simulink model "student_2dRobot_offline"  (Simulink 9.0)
settings: Solver=ode1  StartTime=0.0  StopTime=10  FixedStep=0.002  RelTol=1e-3  AbsTol=1e-6  EnableMultiTasking=on
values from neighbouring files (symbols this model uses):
  K = Am / Beq_v    [d_model_param.m]
  K_AMP = 1    [setup_2d_robot.m]
  K_ENC = 0    [config_srv02.m]
  ki = 0    [setup_2d_robot.m]
  kp = wn^2/K*tau    [d_pv_design.m]    (also in setup_2d_robot.m = 0)
  kv = (-1+2*zeta*wn*tau)/K    [d_pv_design.m]    (also in setup_2d_robot.m = 0)
  Lb_in = 5    [config_2d_robot.m]
  q0 = [0; 0; pi/2; 0]    [setup_2d_robot.m]
  tau = Jeq / Beq_v    [d_model_param.m]
  VMAX_AMP = 0    [config_srv02.m]
  VMAX_DAC = 10    [setup_2d_robot.m]
  wcf = 2 * pi * 50.0    (= 314.159265359)    [setup_2d_robot.m]
  zetaf = 0.9    [setup_2d_robot.m]
undefined symbols (not defined in the file or in its folder): axis_limits, HIL, number_of_trajectories, qc_get_step_size
libraries: quarc_library x4, simulink x2, simulink_extras x2

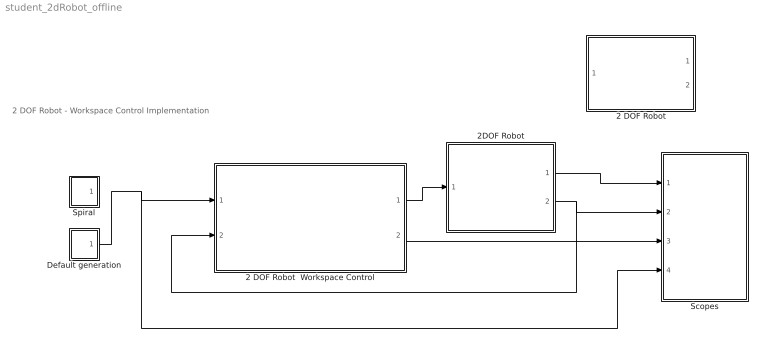
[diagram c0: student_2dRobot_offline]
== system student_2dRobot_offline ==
  note: 2 DOF Robot - Workspace Control Implementation
  2 DOF Robot : Subsystem  Commented=on
  2 DOF Robot  Workspace Control : Subsystem
  2DOF Robot : Subsystem
  Default generation : Subsystem
  Scopes : Subsystem
  Spiral : Subsystem
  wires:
  2 DOF Robot  Workspace Control/1(Reference voltage (V)) -> 2DOF Robot/1(Vi (V))
  Default generation/1(E) -> Scopes/4("Reference [Ex, Ey]"), 2 DOF Robot  Workspace Control/1(Reference [Ex Ey]  (inch))
  2DOF Robot/2(theta_l (rad)) -> Scopes/2(Measured [fi1 fi2]), 2 DOF Robot  Workspace Control/2(Measured [fi1 fi2]  (rad))
  2DOF Robot/1(Vm (V)) -> Scopes/1(Est. motor voltage)
  2 DOF Robot  Workspace Control/2(Reference [fi1 fi2]) -> Scopes/3(Reference [fi1 fi2])

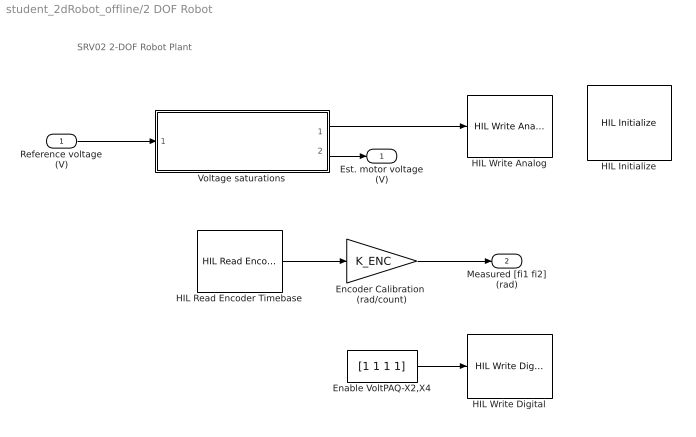
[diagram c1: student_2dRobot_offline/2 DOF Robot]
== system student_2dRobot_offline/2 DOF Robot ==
  note: SRV02 2-DOF Robot Plant
  Reference voltage (V) : Inport
  Enable VoltPAQ-X2,X4 : Constant  Value=[1 1 1 1]
  Encoder Calibration  (rad/count) : Gain  Gain=K_ENC
  HIL Initialize : quarc_library/Data Acquisition/Generic/Configuration/HIL Initialize  object_name=HIL-1  board_type=q8_usb  board_number=0  board_options=update_rate=normal  exclusive=off  active=off  hardware_clocks=[0:2]  clock_modes=[]  initial_clock_frequencies=[]  set_clock_params_at_start=off  set_clock_params_at_switch_in=off  set_clock_frequencies_at_start=off  set_clock_frequencies_at_switch_in=off  analog_input_channels=[0:7]  analog_input_configurations=[]  analog_input_maximums=10  analog_input_minimums=-10  set_analog_input_params_at_start=on  set_analog_input_params_at_switch_in=off  analog_output_channels=[0:7]  analog_output_maximums=10  analog_output_minimums=-10  initial_analog_outputs=[0]  final_analog_outputs=[0]  watchdog_analog_outputs=0  set_analog_output_params_at_start=on  set_analog_output_params_at_switch_in=off  set_analog_outputs_at_start=on  set_analog_outputs_at_switch_in=off  set_analog_outputs_at_terminate=on  set_analog_outputs_at_switch_out=off  set_analog_outputs_on_watchdog=off  digital_input_channels=[]  digital_output_channels=[]  digital_output_configuration=[]  initial_digital_outputs=[1]  final_digital_outputs=[1]  watchdog_digital_outputs=[1]  set_digital_output_params_at_start=off  set_digital_output_params_at_switch_in=off  set_digital_outputs_at_start=on  set_digital_outputs_at_switch_in=off  set_digital_outputs_at_terminate=on  set_digital_outputs_at_switch_out=off  set_digital_outputs_on_watchdog=off  encoder_channels=[0:7]  quadrature=[4]  encoder_filter_frequency=[]  initial_encoder_counts=[0]  set_encoder_params_at_start=on  set_encoder_params_at_switch_in=off  set_encoder_counts_at_start=on  set_encoder_counts_at_switch_in=off  pwm_channels=[]  pwm_modes=[]  pwm_frequency=[]  pwm_configuration=[]  pwm_alignment=[]  pwm_polarity=[]  pwm_leading_deadband=[]  pwm_trailing_deadband=[]  initial_pwm_outputs=[]  final_pwm_outputs=[]  watchdog_pwm_outputs=[]  set_pwm_params_at_start=off  set_pwm_params_at_switch_in=off  set_pwm_outputs_at_start=off  set_pwm_outputs_at_switch_in=off  set_pwm_outputs_at_terminate=off  set_pwm_outputs_at_switch_out=off  set_pwm_outputs_on_watchdog=off  other_output_channels=[]  initial_other_outputs=[]  final_other_outputs=[]  watchdog_other_outputs=[]  set_other_outputs_at_start=off  set_other_outputs_at_switch_in=off  set_other_outputs_at_terminate=off  set_other_outputs_at_switch_out=off  set_other_outputs_on_watchdog=off
  HIL Read Encoder Timebase : quarc_library/Data Acquisition/Generic/Timebases/HIL Read Encoder Timebase  object_name=HIL-1  clock=0  channels=[0:1]  samples_in_buffer=max(ceil(1/qc_get_step_size), 1)  active=on  vector_output=on  data_type_mode=Inherit via back propagation  data_type=double
  HIL Write Analog : quarc_library/Data Acquisition/Generic/Immediate I//O/HIL Write Analog  Tag=unassigned  object_name=HIL-1  channels=[0,1]  sample_time=-1  active=off  vector_input=on
  HIL Write Digital : quarc_library/Data Acquisition/Generic/Immediate I//O/HIL Write Digital  object_name=HIL-1  channels=[0:3]  sample_time=-1  active=off  vector_input=on
  Voltage saturations : Subsystem
  Est. motor voltage (V) : Outport
  Measured [fi1 fi2] (rad) : Outport  Port=2
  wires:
  Enable VoltPAQ-X2,X4/1 -> HIL Write Digital/1
  Encoder Calibration  (rad/count)/1 -> Measured [fi1 fi2] (rad)/1
  Voltage saturations/1(DAQ control voltage  (V)) -> HIL Write Analog/1
  Voltage saturations/2(Estimated  motor voltage (V)) -> Est. motor voltage (V)/1
  Reference voltage (V)/1 -> Voltage saturations/1(Reference voltage (V))
  HIL Read Encoder Timebase/1 -> Encoder Calibration  (rad/count)/1

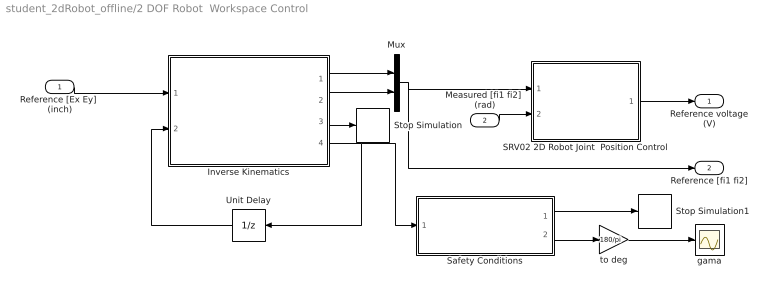
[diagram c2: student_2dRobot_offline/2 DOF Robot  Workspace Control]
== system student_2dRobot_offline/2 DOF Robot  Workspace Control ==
  Reference [Ex Ey]  (inch) : Inport
  Measured [fi1 fi2]  (rad) : Inport  Port=2
  Inverse Kinematics : MATLAB Function  TreatAsAtomicUnit=on
  Mux : Mux  Inputs=2
  SRV02 2D Robot Joint  Position Control : Subsystem
  Safety Conditions : MATLAB Function  TreatAsAtomicUnit=on
  Stop Simulation : Stop
  Stop Simulation1 : Stop
  Unit Delay : UnitDelay  InitialCondition=q0  SampleTime=-1
  gama : Scope
  to deg : Gain  Gain=180/pi
  Reference voltage (V) : Outport
  Reference [fi1 fi2] : Outport  Port=2
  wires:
  Mux/1 -> Reference [fi1 fi2]/1, SRV02 2D Robot Joint  Position Control/1(Reference [fi1 fi2])
  Measured [fi1 fi2]  (rad)/1 -> SRV02 2D Robot Joint  Position Control/2(Measured [f1 fi2])
  SRV02 2D Robot Joint  Position Control/1(Reference voltage (V)) -> Reference voltage (V)/1
  Reference [Ex Ey]  (inch)/1 -> Inverse Kinematics/1(E)
  Inverse Kinematics/1(fi1) -> Mux/1
  Inverse Kinematics/2(fi2) -> Mux/2
  Unit Delay/1 -> Inverse Kinematics/2(q0)
  Inverse Kinematics/4(q) -> Safety Conditions/1(q), Unit Delay/1
  Safety Conditions/1(stop) -> Stop Simulation1/1
  Inverse Kinematics/3(stop) -> Stop Simulation/1
  Safety Conditions/2(gama) -> to deg/1
  to deg/1 -> gama/1

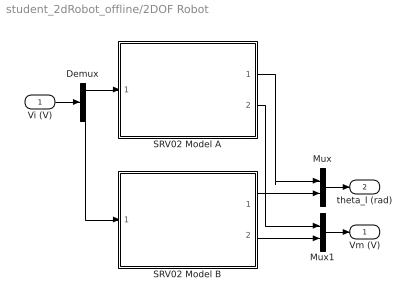
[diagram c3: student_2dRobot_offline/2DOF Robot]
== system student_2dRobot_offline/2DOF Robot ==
  Vi (V) : Inport
  Demux : Demux  Outputs=2
  Mux : Mux  Inputs=2
  Mux1 : Mux  Inputs=2
  SRV02 Model A : Subsystem
  SRV02 Model B : Subsystem
  Vm (V) : Outport
  theta_l (rad) : Outport  Port=2
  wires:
  Demux/1 -> SRV02 Model A/1(Vi (V))
  Demux/2 -> SRV02 Model B/1(Vi (V))
  SRV02 Model A/1(theta_l (rad)) -> Mux/1
  SRV02 Model B/1(theta_l (rad)) -> Mux/2
  SRV02 Model A/2(Vm (V)) -> Mux1/1
  SRV02 Model B/2(Vm (V)) -> Mux1/2
  Vi (V)/1 -> Demux/1
  Mux/1 -> theta_l (rad)/1
  Mux1/1 -> Vm (V)/1

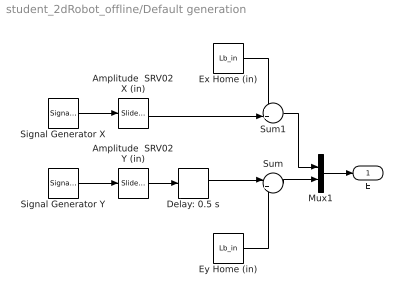
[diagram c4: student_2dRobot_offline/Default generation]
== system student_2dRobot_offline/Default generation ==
  Amplitude  SRV02 X (in) : simulink/Math Operations/Slider Gain  gain=0.500  low=0  high=1
  Amplitude  SRV02 Y (in) : simulink/Math Operations/Slider Gain  gain=0.5  low=0  high=1
  Delay: 0.5 s : TransportDelay  DelayTime=0.5  FixedBuffer=on
  Ex Home (in) : Constant  Value=Lb_in
  Ey Home (in) : Constant  Value=Lb_in
  Mux1 : Mux  Inputs=2
  Signal Generator X : SignalGenerator  WaveForm=square  Frequency=0.5
  Signal Generator Y : SignalGenerator  WaveForm=square  Frequency=0.5
  Sum : Sum  Inputs=|++
  Sum1 : Sum  Inputs=++|
  E : Outport
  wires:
  Delay: 0.5 s/1 -> Sum/1
  Ey Home (in)/1 -> Sum/2
  Ex Home (in)/1 -> Sum1/1
  Amplitude  SRV02 X (in)/1 -> Sum1/2
  Amplitude  SRV02 Y (in)/1 -> Delay: 0.5 s/1
  Sum/1 -> Mux1/2
  Signal Generator Y/1 -> Amplitude  SRV02 Y (in)/1
  Sum1/1 -> Mux1/1
  Signal Generator X/1 -> Amplitude  SRV02 X (in)/1
  Mux1/1 -> E/1

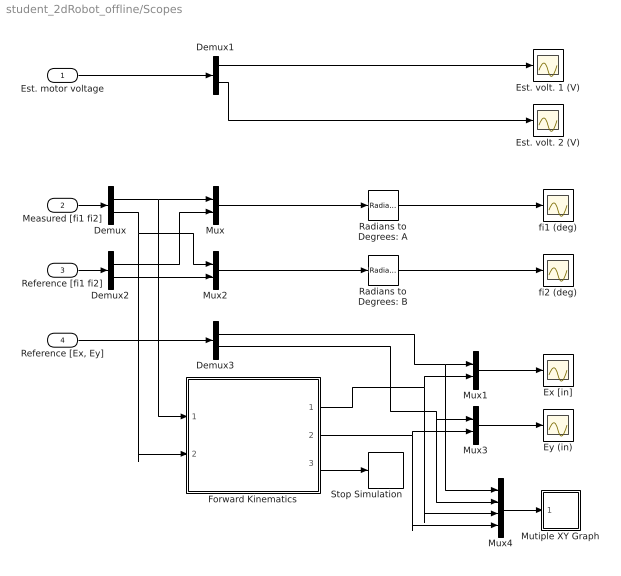
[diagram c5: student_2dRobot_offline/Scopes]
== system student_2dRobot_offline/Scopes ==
  Est. motor voltage : Inport
  Measured [fi1 fi2] : Inport  Port=2
  Reference [fi1 fi2] : Inport  Port=3
  "Reference [Ex, Ey]" : Inport  Port=4
  Demux{,1..3} (4 alike) : Demux  Outputs=2
  Est. volt. 1 (V) : Scope
  Est. volt. 2 (V) : Scope
  Ex [in] : Scope
  Ey (in) : Scope
  Forward Kinematics : MATLAB Function  TreatAsAtomicUnit=on
  Mutiple XY Graph : Subsystem
  Mux{,1..3} (4 alike) : Mux  Inputs=2
  Mux4 : Mux
  Radians to Degrees: A : simulink_extras/Transformations/Radians to Degrees
  Radians to Degrees: B : simulink_extras/Transformations/Radians to Degrees
  Stop Simulation : Stop
  fi1 (deg) : Scope
  fi2 (deg) : Scope
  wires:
  Demux/1 -> Mux/1, Forward Kinematics/1(fi1)
  Demux/2 -> Forward Kinematics/2(fi2), Mux2/1
  Mux2/1 -> Radians to Degrees: B/1
  Mux/1 -> Radians to Degrees: A/1
  Demux1/1 -> Est. volt. 1 (V)/1
  Demux1/2 -> Est. volt. 2 (V)/1
  Measured [fi1 fi2]/1 -> Demux/1
  Est. motor voltage/1 -> Demux1/1
  Radians to Degrees: A/1 -> fi1 (deg)/1
  Radians to Degrees: B/1 -> fi2 (deg)/1
  Reference [fi1 fi2]/1 -> Demux2/1
  Mux1/1 -> Ex [in]/1
  Mux3/1 -> Ey (in)/1
  "Reference [Ex, Ey]"/1 -> Demux3/1
  Demux3/2 -> Mux4/2, Mux3/1
  Demux3/1 -> Mux4/1, Mux1/1
  Forward Kinematics/1(Ex) -> Mux4/3, Mux1/2
  Forward Kinematics/2(Ey) -> Mux4/4, Mux3/2
  Forward Kinematics/3(stop) -> Stop Simulation/1
  Demux2/1 -> Mux/2
  Demux2/2 -> Mux2/2
  Mux4/1 -> Mutiple XY Graph/1(In1)

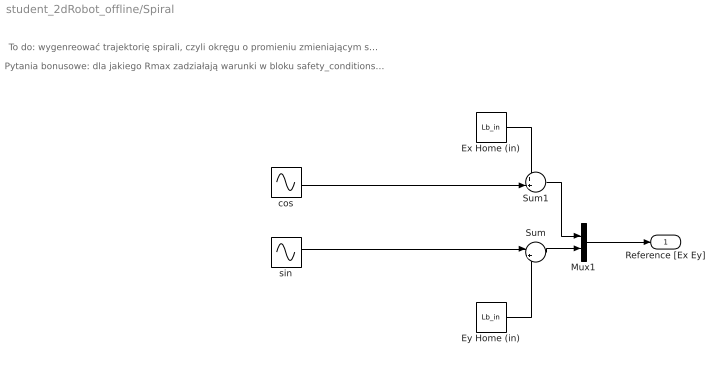
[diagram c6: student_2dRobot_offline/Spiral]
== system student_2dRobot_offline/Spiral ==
  note: Pytania bonusowe: dla jakiego Rmax zadziałają warunki w bloku safety_conditions? Jak wygenerować krzywe Lissajous? (https://pl.m.wikipedia.org/wiki/Krzywa_Lissajous)
  note: To do: wygenreować trajektorię spirali, czyli okręgu o promieniu zmieniającym się od r=0 do r=Rmax w pewnym przedziale czasowym
  Ex Home (in) : Constant  Value=Lb_in
  Ey Home (in) : Constant  Value=Lb_in
  Mux1 : Mux  Inputs=2
  Sum : Sum  Inputs=|++
  Sum1 : Sum  Inputs=++|
  cos : Sin  Phase=pi/2  SampleTime=0
  sin : Sin  SampleTime=0
  Reference [Ex Ey] : Outport
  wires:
  sin/1 -> Sum/1
  Ey Home (in)/1 -> Sum/2
  Ex Home (in)/1 -> Sum1/1
  cos/1 -> Sum1/2
  Sum/1 -> Mux1/2
  Sum1/1 -> Mux1/1
  Mux1/1 -> Reference [Ex Ey]/1

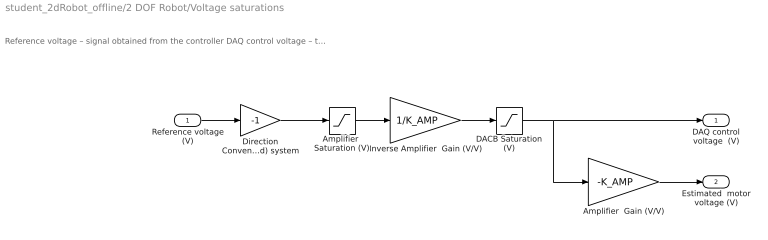
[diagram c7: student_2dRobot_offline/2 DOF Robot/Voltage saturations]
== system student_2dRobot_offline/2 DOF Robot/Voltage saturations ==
  note: Reference voltage – signal obtained from the controller DAQ control voltage – the voltage that can be realised by the hardware (saturations are taken into account) Estimated motor voltage – the input motor voltage after going through the DAQ board and amplifier limitiations (assuming ideal amplifier characteristics)
  Reference voltage (V) : Inport
  Amplifier  Gain (V/V) : Gain  Gain=-K_AMP
  Amplifier  Saturation (V) : Saturate  UpperLimit=VMAX_AMP  LowerLimit=-VMAX_AMP
  DACB Saturation (V) : Saturate  UpperLimit=VMAX_DAC  LowerLimit=-VMAX_DAC
  Direction Convention: (Right-Hand) system : Gain  Gain=-1
  Inverse Amplifier  Gain (V/V) : Gain  Gain=1/K_AMP
  DAQ control voltage  (V) : Outport
  Estimated  motor voltage (V) : Outport  Port=2
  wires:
  Amplifier  Saturation (V)/1 -> Inverse Amplifier  Gain (V/V)/1
  Reference voltage (V)/1 -> Direction Convention: (Right-Hand) system/1
  Inverse Amplifier  Gain (V/V)/1 -> DACB Saturation (V)/1
  DACB Saturation (V)/1 -> Amplifier  Gain (V/V)/1, DAQ control voltage  (V)/1
  Amplifier  Gain (V/V)/1 -> Estimated  motor voltage (V)/1
  Direction Convention: (Right-Hand) system/1 -> Amplifier  Saturation (V)/1

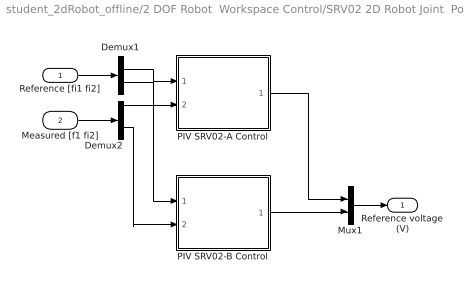
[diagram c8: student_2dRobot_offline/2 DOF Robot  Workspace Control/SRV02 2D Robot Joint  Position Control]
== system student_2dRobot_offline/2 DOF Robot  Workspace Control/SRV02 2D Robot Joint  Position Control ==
  Reference [fi1 fi2] : Inport
  Measured [f1 fi2] : Inport  Port=2
  Demux1 : Demux  Outputs=2
  Demux2 : Demux  Outputs=2
  Mux1 : Mux  Inputs=2
  PIV SRV02-A Control : Subsystem
  PIV SRV02-B Control : Subsystem
  Reference voltage (V) : Outport
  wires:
  PIV SRV02-A Control/1(Ref. voltage 1) -> Mux1/1
  PIV SRV02-B Control/1(Ref. voltage 2) -> Mux1/2
  Demux2/1 -> PIV SRV02-A Control/2(Measured fi1)
  Demux2/2 -> PIV SRV02-B Control/2(Measured fi2)
  Measured [f1 fi2]/1 -> Demux2/1
  Mux1/1 -> Reference voltage (V)/1
  Reference [fi1 fi2]/1 -> Demux1/1
  Demux1/1 -> PIV SRV02-A Control/1(Reference fi1)
  Demux1/2 -> PIV SRV02-B Control/1(Reference fi2)

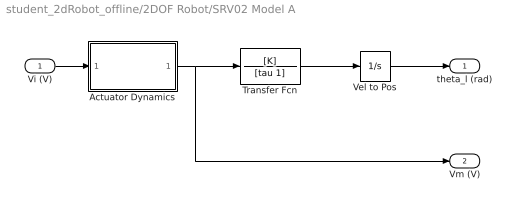
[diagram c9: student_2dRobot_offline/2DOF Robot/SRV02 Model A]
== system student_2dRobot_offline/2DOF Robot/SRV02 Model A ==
  Vi (V) : Inport
  Actuator Dynamics : Subsystem
  Transfer Fcn : TransferFcn  Numerator=[K]  Denominator=[tau 1]
  Vel to Pos : Integrator
  theta_l (rad) : Outport
  Vm (V) : Outport  Port=2
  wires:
  Vi (V)/1 -> Actuator Dynamics/1(Vi (V))
  Actuator Dynamics/1(Vm (V)) -> Vm (V)/1, Transfer Fcn/1
  Transfer Fcn/1 -> Vel to Pos/1
  Vel to Pos/1 -> theta_l (rad)/1

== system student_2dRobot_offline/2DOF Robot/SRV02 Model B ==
  Vi (V) : Inport
  Actuator Dynamics : Subsystem
  Transfer Fcn : TransferFcn  Numerator=[K]  Denominator=[tau 1]
  Vel to Pos : Integrator
  theta_l (rad) : Outport
  Vm (V) : Outport  Port=2
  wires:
  Transfer Fcn/1 -> Vel to Pos/1
  Vel to Pos/1 -> theta_l (rad)/1
  Actuator Dynamics/1(Vm (V)) -> Transfer Fcn/1, Vm (V)/1
  Vi (V)/1 -> Actuator Dynamics/1(Vi (V))

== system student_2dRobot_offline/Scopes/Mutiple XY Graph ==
  In1 : Inport
  Level-2 MATLAB S-Function : M-S-Function  FunctionName=multiple_xy_graph  Parameters=number_of_trajectories,axis_limits
  Rate Transition : RateTransition  OutPortSampleTime=sample_time
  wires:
  Rate Transition/1 -> Level-2 MATLAB S-Function/1
  In1/1 -> Rate Transition/1

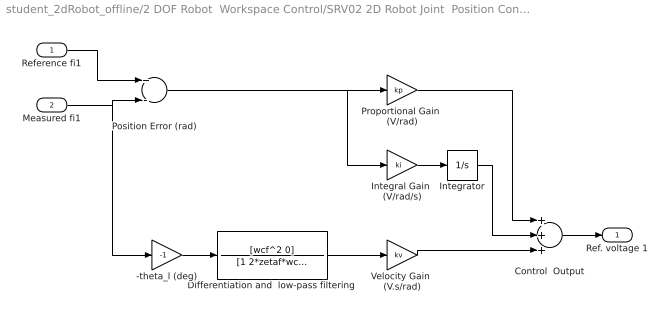
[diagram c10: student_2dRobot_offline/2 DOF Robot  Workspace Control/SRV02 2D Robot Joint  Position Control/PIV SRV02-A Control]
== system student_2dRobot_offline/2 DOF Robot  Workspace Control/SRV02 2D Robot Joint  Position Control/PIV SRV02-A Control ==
  Reference fi1 : Inport
  Measured fi1 : Inport  Port=2
  -theta_l (deg) : Gain  Gain=-1
  Control  Output : Sum  Inputs=+++
  Differentiation and  low-pass filtering : TransferFcn  Numerator=[wcf^2 0]  Denominator=[1 2*zetaf*wcf wcf^2]
  Integral Gain  (V/rad/s) : Gain  Gain=ki
  Integrator : Integrator  LimitOutput=on  UpperSaturationLimit=VMAX_DAC  LowerSaturationLimit=-VMAX_DAC
  Position Error (rad) : Sum  Inputs=+-
  Proportional Gain  (V/rad) : Gain  Gain=kp
  Velocity Gain  (V.s/rad) : Gain  Gain=kv
  Ref. voltage 1 : Outport
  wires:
  Integrator/1 -> Control  Output/2
  Velocity Gain  (V.s/rad)/1 -> Control  Output/3
  Integral Gain  (V/rad/s)/1 -> Integrator/1
  -theta_l (deg)/1 -> Differentiation and  low-pass filtering/1
  Position Error (rad)/1 -> Proportional Gain  (V/rad)/1, Integral Gain  (V/rad/s)/1
  Measured fi1/1 -> -theta_l (deg)/1, Position Error (rad)/2
  Control  Output/1 -> Ref. voltage 1/1
  Proportional Gain  (V/rad)/1 -> Control  Output/1
  Differentiation and  low-pass filtering/1 -> Velocity Gain  (V.s/rad)/1
  Reference fi1/1 -> Position Error (rad)/1

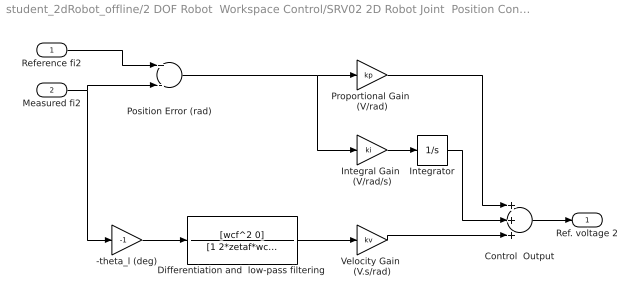
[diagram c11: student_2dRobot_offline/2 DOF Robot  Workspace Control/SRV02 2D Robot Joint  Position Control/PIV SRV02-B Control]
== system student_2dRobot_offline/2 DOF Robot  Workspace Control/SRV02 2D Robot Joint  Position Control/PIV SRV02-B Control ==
  Reference fi2 : Inport
  Measured fi2 : Inport  Port=2
  -theta_l (deg) : Gain  Gain=-1
  Control  Output : Sum  Inputs=+++
  Differentiation and  low-pass filtering : TransferFcn  Numerator=[wcf^2 0]  Denominator=[1 2*zetaf*wcf wcf^2]
  Integral Gain  (V/rad/s) : Gain  Gain=ki
  Integrator : Integrator  LimitOutput=on  UpperSaturationLimit=VMAX_DAC  LowerSaturationLimit=-VMAX_DAC
  Position Error (rad) : Sum  Inputs=+-
  Proportional Gain  (V/rad) : Gain  Gain=kp
  Velocity Gain  (V.s/rad) : Gain  Gain=kv
  Ref. voltage 2 : Outport
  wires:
  Differentiation and  low-pass filtering/1 -> Velocity Gain  (V.s/rad)/1
  Proportional Gain  (V/rad)/1 -> Control  Output/1
  Reference fi2/1 -> Position Error (rad)/1
  Control  Output/1 -> Ref. voltage 2/1
  Measured fi2/1 -> Position Error (rad)/2, -theta_l (deg)/1
  Position Error (rad)/1 -> Integral Gain  (V/rad/s)/1, Proportional Gain  (V/rad)/1
  -theta_l (deg)/1 -> Differentiation and  low-pass filtering/1
  Integral Gain  (V/rad/s)/1 -> Integrator/1
  Velocity Gain  (V.s/rad)/1 -> Control  Output/3
  Integrator/1 -> Control  Output/2

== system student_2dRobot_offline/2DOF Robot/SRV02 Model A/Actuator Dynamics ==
  note: Actuator Dynamics: Vi is the ideal voltage and Vm is the input motor voltage after going through the DAC board and amplifier limitiations.
  Vi (V) : Inport
  Amplifier  Gain (V/V) : Gain  Gain=K_AMP
  Amplifier  Saturation (V) : Saturate  UpperLimit=VMAX_AMP  LowerLimit=-VMAX_AMP
  DACB Saturation (V) : Saturate  UpperLimit=VMAX_DAC  LowerLimit=-VMAX_DAC
  Inverse Amplifier  Gain (V/V) : Gain  Gain=1/K_AMP
  Vm (V) : Outport
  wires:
  Amplifier  Saturation (V)/1 -> Vm (V)/1
  Vi (V)/1 -> Inverse Amplifier  Gain (V/V)/1
  Amplifier  Gain (V/V)/1 -> Amplifier  Saturation (V)/1
  DACB Saturation (V)/1 -> Amplifier  Gain (V/V)/1
  Inverse Amplifier  Gain (V/V)/1 -> DACB Saturation (V)/1

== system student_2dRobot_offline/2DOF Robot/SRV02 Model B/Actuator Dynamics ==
  note: Actuator Dynamics: Vi is the ideal voltage and Vm is the input motor voltage after going through the DAC board and amplifier limitiations.
  Vi (V) : Inport
  Amplifier  Gain (V/V) : Gain  Gain=K_AMP
  Amplifier  Saturation (V) : Saturate  UpperLimit=VMAX_AMP  LowerLimit=-VMAX_AMP
  DACB Saturation (V) : Saturate  UpperLimit=VMAX_DAC  LowerLimit=-VMAX_DAC
  Inverse Amplifier  Gain (V/V) : Gain  Gain=1/K_AMP
  Vm (V) : Outport
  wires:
  Amplifier  Saturation (V)/1 -> Vm (V)/1
  Vi (V)/1 -> Inverse Amplifier  Gain (V/V)/1
  Amplifier  Gain (V/V)/1 -> Amplifier  Saturation (V)/1
  DACB Saturation (V)/1 -> Amplifier  Gain (V/V)/1
  Inverse Amplifier  Gain (V/V)/1 -> DACB Saturation (V)/1

== matlab function 2 DOF Robot 
Workspace Control/Inverse Kinematics ==
% SRV02 2D Robot Inverse Kinematics
% Computes the servo angles required to achieve the given
% end-effector global  Cartesian coordinates.
%
% Input parameters:
% Ex        End-effector global Cartesian x-axis coordinate     (in)
% Ey        End-effector global Cartesian y-axis coordinate     (in)
% Lb_in     Link length                                         (in)
%
% Output parameters:
% theta_A   Servo A angle to get (Ex,Ey)   (rad)
% theta_B   Servo B angle to get (Ex,Ey)   (rad)
%
function [fi1, fi2, stop, q] = inv_kin_2d_robot(E, q0, Lb_in)
% q == [fi1, fi2, alfa, beta]'

% TO DO: wyliczyc q na podstawie q0 oraz punktu E

end

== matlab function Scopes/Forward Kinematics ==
% SRV02 2D Robot Forward Kinematics
% Computes the location of the end-effector in global Cartesian 
% coordinates given the servo angles.
%
% Input parameters:
% theta_A   Measured servo A angle                              (rad)
% theta_B   Measured servo B angle                              (rad)
% Lb_in     Link length                                         (in)
%
% Output parameters:
% Ex        End-effector global Cartesian x-axis coordinate     (in)
% Ey        End-effector global Cartesian y-axis coordinate     (in)
%
function [Ex,Ey, stop] = fwrd_kin_2d_robot(fi1, fi2, Lb_in)
% q == [fi1, fi2, alfa, beta]'

% TO DO: wyliczyc E na podstawie fi, fi2

stop = 0;
E = zeros(2,1);
Ex = E(1);
Ey = E(2);
end


function R = R(fi)
R = [cos(fi), -sin(fi); sin(fi), cos(fi)];
end

== matlab function 2 DOF Robot 
Workspace Control/Safety Conditions ==
% Safety conditions for Quanser 2 dof robot

% stop - flag to stop the simulation if sefety conditions are not met
% gama - angle between links 2 and 3 (for debugging purposes)
% settable parameters: safety angle, TOL

% Note that Lb_in is a parameter (check Editor tab -> Edit Data)

function [stop, gama] = safety_conditions(q, Lb_in)
safety_angle = pi / 6; % rad
TOL = 1.75; % [inch] Niedopuszczalna odleglosc od srodkow serwomechanizmow 
            %        (przyjeta arbitralnie)

% to do: napisać warunki dla awaryjnego stopu układu
% - dla położenia punktu E
% - dla wartości kąta gamma



if beta < 0
    gama = beta + pi - alfa; % -pi < beta < pi
else
    gama = beta - pi - alfa; % 0 < beta < 2*pi (zob. instrukcja)
end
